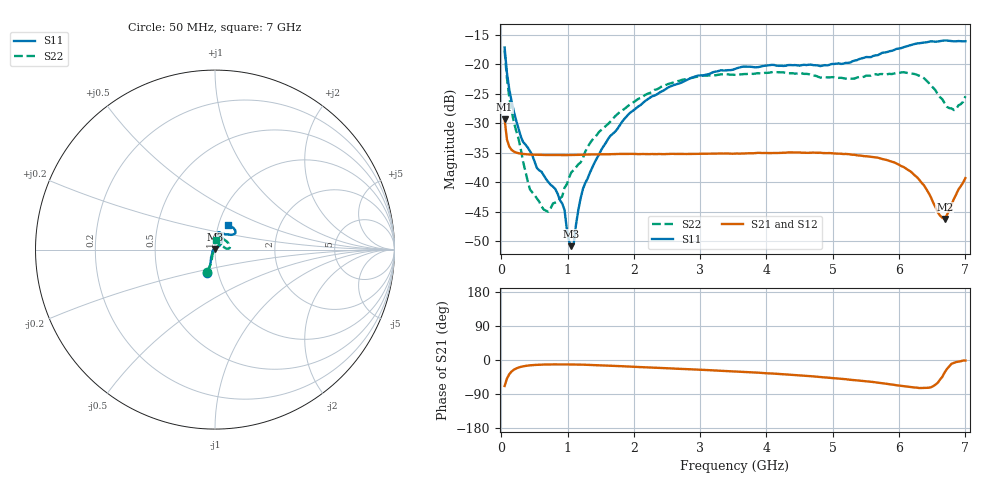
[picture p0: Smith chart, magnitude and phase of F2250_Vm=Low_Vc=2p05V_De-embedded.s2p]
! Integrated Device Technology
! Corporate Headquarters
! 6024 Silver Creek Valley Road
! San Jose, CA 95138  USA
! Phone:  1-408-284-8200
! Toll Free:  1-800-223-1366
! Webpage:  http://www.idt.com/
! Timing and RF Division
! 515 Groton Road, Suite 102
! Westford, MA 01886-6024
! Device:  F2250
! Description: Voltage Variable RF Attenuator
! Frequency:  50.0 -  6000.00 MHz
! Package:  3x3 mm Thin QFN Plastic Package: 16 pin
! Ports:  2 RF, 3 DC
!  Pin  1  = GND
!  Pin  2  = NC
!  Pin  3  = RF1  = Port 1
!  Pin  4  = NC
!  Pin  5  = GND
!  Pin  6  = GND
!  Pin  7  = GND
!  Pin  8  = GND
!  Pin  9  = NC
!  Pin 10  = RF2  = Port 2
!  Pin 11  = NC
!  Pin 12  = GND
!  Pin 13  = GND
!  Pin 14  = VCNTRL
!  Pin 15  = VDD
!  Pin 16  = VMODE
! Vcntrl:  2.050 Volts
! Vmode:  +0.000 Volts
! Vdd:  +3.30  Volts
! Current:  1.181 mA
! Data:  The device was measured on a the F2250 evaluation board which has
!  individual transmission lines to the RF pins.  Data was collected
!  using a calibrated network analyzer.  The evaluation board was
!  de-embedded using a TRL calibration technique.
!  The reference plane is the edge of the package pin.
! Misc:  SN 10
!  Action Tracker AT0258
! Date Measured:  2014-11-26
! Date:  2015-10-15  MJV
! Note:
!  Integrated Device Technology supplies this data as a sample of measured
!  data at the package pin for this product.  Your particular data for this
!  product may vary.
!  Data was taken at 25 degrees C.
!  Integrated Device Technology reserves the right to change this data at anytime.
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# GHz S dB R 50
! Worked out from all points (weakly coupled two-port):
!   201 points, 50 MHz to 7 GHz, reference 50 ohm
!   highest |S21| = -29.31 dB at 50 MHz (marker M1); lowest = -46.2 dB at 6.687 GHz (marker M2)
!   lowest |S11| = -50.8 dB at 1.058 GHz (marker M3), VSWR 1.01, Z = 49.8 + j0.24 ohm
!   |S11| at or under -10 dB: start of sweep to end of sweep
!   |S22| runs from -45.0 to -17.7 dB; largest |S21 - S12| = 6.3e-05
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0.05  -17.18 -108.6  -29.31 -68.6  -29.31 -68.6  -17.66 -109.1
0.08475  -21.45 -107.4  -32.72 -49.3  -32.72 -49.3  -22.30 -105.5
0.189  -28.01 -119.6  -34.79 -25.7  -34.79 -25.7  -29.79 -115.8
0.29325  -32.20 -127.7  -35.15 -18.1  -35.15 -18.1  -34.33 -120.4
0.43225  -34.71 -144.6  -35.30 -14.1  -35.29 -14.1  -41.20 -153.0
0.71025  -39.97 -168.4  -35.38 -11.8  -35.38 -11.8  -44.98 136.0
0.9535  -44.66 170.2  -35.39 -11.7  -35.39 -11.7  -40.93 99.4
1.023  -49.99 143.9  -35.39 -11.8  -35.38 -11.7  -39.17 80.7
1.05775  -50.81 123.1  -35.38 -11.8  -35.38 -11.8  -38.27 77.0
1.0925  -50.41 88.5  -35.37 -11.9  -35.37 -11.9  -37.93 72.5
1.162  -44.69 56.6  -35.35 -12.1  -35.35 -12.1  -36.96 62.5
1.2315  -41.11 44.1  -35.33 -12.3  -35.32 -12.3  -35.86 55.7
1.3705  -37.53 38.6  -35.28 -13.2  -35.28 -13.2  -32.84 51.1
1.6485  -32.10 42.0  -35.24 -15.0  -35.24 -15.0  -29.69 49.8
2.37825  -24.87 47.3  -35.21 -20.8  -35.21 -20.8  -24.09 49.2
3.525  -20.80 72.5  -35.15 -30.2  -35.15 -30.2  -21.81 70.9
4.7065  -20.17 72.3  -34.97 -43.3  -34.97 -43.3  -21.92 70.1
5.85325  -17.82 40.4  -36.38 -63.8  -36.38 -63.9  -21.64 18.9
6.33975  -16.40 41.0  -40.08 -73.9  -40.09 -73.9  -22.13 4.8
6.68725  -15.99 48.8  -46.22 -32.6  -46.21 -32.2  -26.63 25.0
6.82625  -16.14 53.6  -42.81 -7.6  -42.76 -7.7  -27.77 52.7
7  -16.12 63.2  -39.29 -1.4  -39.25 -1.4  -25.43 86.2
